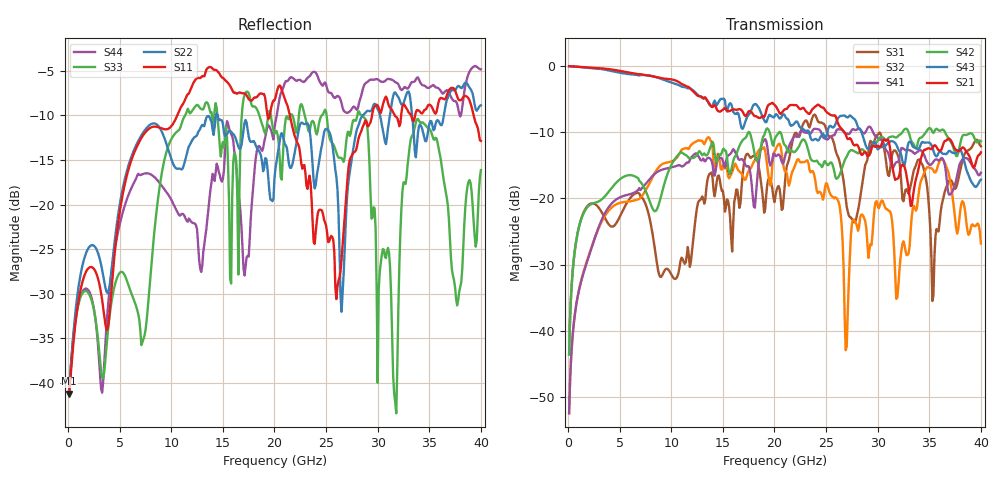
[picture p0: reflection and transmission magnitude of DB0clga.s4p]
! ADC12DJ3200QML-SP
! 196-pin ZMX package
! CLGA Ceramic Package without columns (ceramic land grid array)
! Texas Instruments 4/21/2021
! Single-ended  S-parameters
! PORT#  PORT_NAME  NET_NAME
! PORT1:  DAxN.DIEBUMP DAxN
! PORT2:  DAxN.BGA  DAxN
! PORT3:  DAxP.DIEBUMP DAxP
! PORT4:  DAxP.BGA  DAxP
! Touchstone Ver. 1.0
! Number of ports is 4
# Hz	S	MA	R	50.000000
! SCATTERING PARAMETERS  :
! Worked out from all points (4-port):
!   400 points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, 100 MHz to 40 GHz, reference 50 ohm
!   strongest paths, dB at 100 MHz, 10.1 GHz, 20.1 GHz, 30.1 GHz, 40 GHz:
!     S21: -0.1, -2.1, -6.1, -12.2, -13.1
!     S43: -0.1, -2.6, -7.4, -12.5, -17.2
!     S42: -43.6, -14.7, -10.8, -11.0, -11.4
!     S41: -52.4, -15.3, -13.6, -11.1, -16.1
!     S32: -52.4, -14.4, -12.7, -21.5, -26.8
!     S31: -43.5, -31.8, -19.6, -10.2, -12.2
!   lowest |S11| = -41.2 dB at 100 MHz (marker M1), VSWR 1.02, Z = 50.8 - j0.261 ohm
!   |S11| at or under -10 dB: start of sweep to 10.58 GHz; 21.48 GHz to 29.45 GHz (7.965 GHz wide, 31.3 % of centre); 39.3 GHz to end of sweep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
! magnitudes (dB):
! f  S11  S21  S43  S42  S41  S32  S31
! 100 MHz  -41.2  -0.1  -0.1  -43.6  -52.4  -52.4  -43.5
! 12.6 GHz  -5.8  -4.6  -4.5  -13.2  -13.6  -11.3  -20.6
! 26.5 GHz  -26.1  -9.5  -7.6  -15.6  -9.7  -23.8  -15.8
! 28.8 GHz  -10.6  -13.0  -11.8  -13.1  -10.1  -23.5  -14.9
! 31.8 GHz  -10.2  -17.1  -11.9  -10.8  -14.6  -35.2  -13.0
! 33.8 GHz  -9.4  -16.6  -12.5  -12.2  -13.1  -21.5  -14.6
! 40 GHz  -12.9  -13.1  -17.2  -11.4  -16.1  -26.8  -12.2
